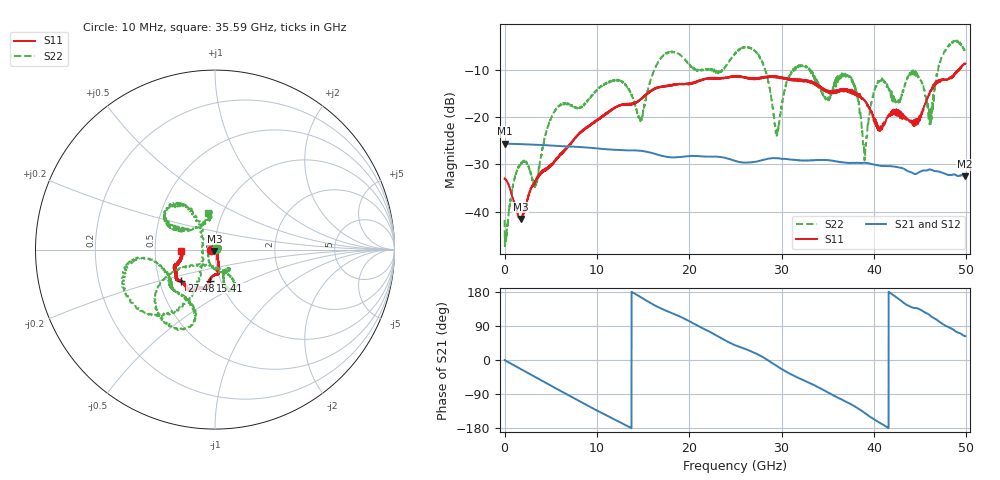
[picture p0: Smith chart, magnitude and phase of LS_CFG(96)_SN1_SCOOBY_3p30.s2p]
!Keysight Technologies,N5245B,MY58422026,A.13.80.08
!Date: Thursday, March 19, 2020 23:57:14
!Correction: S11(Full 2 Port(1,2))
!S21(Full 2 Port(1,2))
!S12(Full 2 Port(1,2))
!S22(Full 2 Port(1,2))
!S2P File: Measurements: S11, S21, S12, S22:
# Hz S DB R 50.0
!freq dBS11 angS11 dBS21 angS21 dBS12 angS12 dBS22 angS22
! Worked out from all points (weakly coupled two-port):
!   4991 points, 10 MHz to 49.91 GHz, reference 50 ohm
!   highest |S21| = -25.58 dB at 20 MHz (marker M1); lowest = -32.5 dB at 49.83 GHz (marker M2)
!   lowest |S11| = -41.6 dB at 1.77 GHz (marker M3), VSWR 1.02, Z = 49.7 - j0.774 ohm
!   |S11| at or under -10 dB: start of sweep to 49.12 GHz; 49.16853 GHz to 49.22373 GHz (55.2 MHz wide, 0.112 % of centre)
!   |S22| runs from -47.3 to -3.7 dB; largest |S21 - S12| = 0.00049
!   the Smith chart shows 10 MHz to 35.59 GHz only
!   S11 on the Smith chart (normalised r, x): 10 MHz: 0.96, -0.01; 15.41 GHz: 0.89, -0.32; 27.48 GHz: 0.65, -0.24; 35.59 GHz: 0.68, -0.01
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1e7  -33.04 -173.0  -25.58 -0.3  -25.56 -0.4  -41.77 6.3
2e7  -32.93 -178.1  -25.58 -0.4  -25.57 -0.4  -45.66 -3.7
1.77e9  -41.59 -110.8  -25.70 -24.1  -25.70 -24.0  -29.83 5.3
3.33e9  -33.42 -59.5  -25.83 -45.0  -25.82 -44.9  -34.27 130.8
5.38e9  -29.26 -63.1  -26.04 -72.6  -26.03 -72.6  -18.90 -87.9
8.33e9  -23.20 -75.0  -26.34 -111.5  -26.34 -111.4  -17.79 -63.1
1.541e10  -15.12 -99.3  -27.32 156.2  -27.31 156.3  -15.30 -146.8
1.665e10  -13.73 -100.5  -27.97 139.4  -27.96 139.5  -8.26 -145.5
2.496e10  -11.40 -125.9  -29.21 39.2  -29.20 39.4  -6.56 -171.0
2.748e10  -11.86 -137.0  -29.33 14.1  -29.33 14.4  -6.73 -127.9
2.947e10  -11.33 -142.7  -28.69 -15.8  -28.68 -15.4  -23.43 -175.7
3.103e10  -11.93 -149.7  -28.99 -37.8  -29.00 -37.6  -10.41 125.7
3.328e10  -12.56 -159.9  -29.12 -63.7  -29.13 -63.3  -10.63 153.2
3.559e10  -14.39 -178.2  -29.28 -93.1  -29.22 -92.6  -13.61 101.5
3.77e10  -15.02 172.2  -29.68 -119.3  -29.60 -119.4  -12.18 131.7
3.902e10  -16.43 169.8  -29.65 -139.9  -29.63 -140.1  -28.38 -114.0
4.021e10  -21.70 156.7  -30.10 -159.5  -30.09 -159.7  -13.46 -8.9
4.16e10  -19.48 101.2  -30.37 179.9  -30.39 180.0  -14.16 22.4
4.614e10  -14.43 5.5  -31.07 116.4  -31.08 116.6  -21.46 -51.1
4.749e10  -12.03 7.2  -31.82 94.3  -31.83 94.5  -6.71 -81.4
4.983e10  -8.62 -14.6  -32.50 63.2  -32.51 63.4  -5.90 -27.0
4.991e10  -8.59 -13.7  -32.50 62.9  -32.52 62.9  -6.28 -28.7
